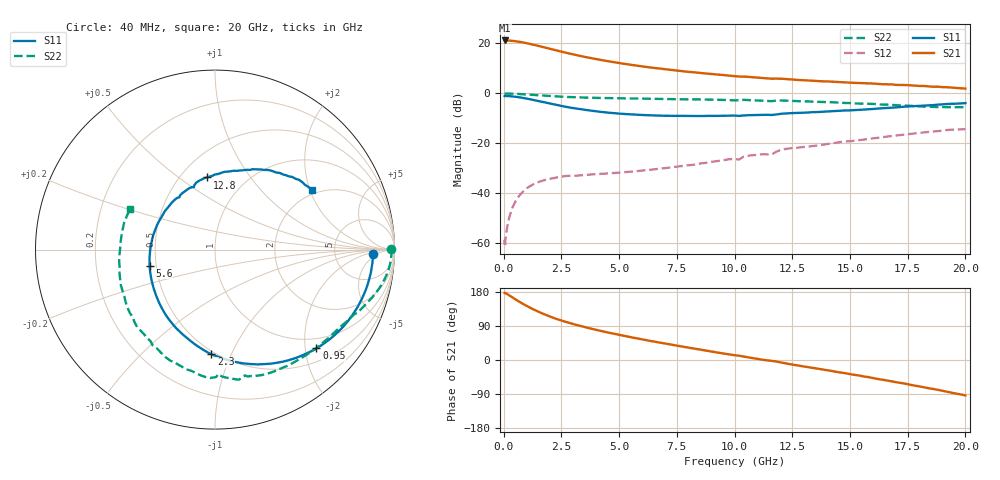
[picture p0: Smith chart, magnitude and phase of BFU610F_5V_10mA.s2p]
! Filename:  P:\Prog\Test\Noise\ATS_data\Testdata_Net\SplitFiles\BFU610_2W_A5_HighFreq_5V_10mA_D.s2p
! Date/Time: Wed 10/Aug/2011 16:58:24
! BFU610_2W_A5_HighFreq_5V_1mA_10mA_Bias4_R.s2p
! MDIF S-parameter v. bias file
! BFU610_2W_A5_HighFreq_5V_1mA_10mA
! Date/time Mon Aug 08 14:15:19 2011
! VAR V_out= 5.0010
! VAR I_out= 9.9950
! VAR V_in= 0.8863
! VAR I_in= 0.0857
! Device data file deembeded for feedlines and parallel
! Original file: \SplitFiles\BFU610_2W_A5_HighFreq_5V_10mA_R.s2p
! Feed-files: PR003V01_101208_Feed1.s2p, PR003V01_101208_Feed2.s2p
! Parallel-file: PR003V01_101208_Par.s2p
# MHz S MA R 50
!  Freq-MHz  S11-mag  S11-arg  S21-mag  S21-arg  S12-mag  S12-arg  S22-mag  S22-arg
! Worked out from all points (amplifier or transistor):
!   167 points, 40 MHz to 20 GHz, reference 50 ohm
!   highest |S21| = 21.1 dB at 40 MHz (marker M1)
!   |S21| within 3 dB of that: start of sweep to 1.861 GHz
!   unconditionally stable (mu >= 1): start of sweep to 59.98 MHz; 3.421 GHz to 17.92 GHz
!   at 550 MHz: K = 0.21, MSG = 31.8 dB, |S12| = -42.7 dB
!   at 4.2 GHz: K = 1.21, MAG = 20.0 dB, |S12| = -32.3 dB
!   at 20 GHz: K = 0.89, MSG = 8.1 dB, |S12| = -14.4 dB
!   S11 on the Smith chart (normalised r, x): 40 MHz: 15, -4; 950 MHz: 0.77, -2.24; 2.3 GHz: 0.48, -0.84; 5.6 GHz: 0.46, -0.10; 12.8 GHz: 0.67, +0.64; 20 GHz: 1.84, +2.06
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40  0.8803 -1.8  11.38 177.2  0.0009164 41.6  0.9799 0.1
50  0.8721 -2.4  11.33 177.4  0.001163 22.7  0.9814 -0.2
140  0.8785 -6.8  11.32 174.4  0.001962 68.5  0.9832 -1.7
260  0.8728 -12.7  11.3 169.7  0.003489 74.4  0.9815 -3.4
400  0.8613 -19.4  11.16 164.2  0.005391 74.8  0.9773 -5.3
650  0.8334 -31.1  10.78 154.8  0.008555 71.0  0.9656 -8.6
950  0.7887 -44.2  10.15 144.2  0.01196 64.8  0.9473 -12.1
1200  0.7482 -54.4  9.569 136.3  0.01433 60.1  0.9302 -14.7
1500  0.6985 -65.8  8.87 127.5  0.01664 55.1  0.9107 -17.6
1850  0.6443 -77.9  8.081 118.3  0.01874 50.4  0.8889 -20.6
2300  0.5826 -92.0  7.139 108.2  0.02065 46.5  0.8619 -24.4
2900  0.5136 -108.4  6.14 96.7  0.02223 40.6  0.8381 -28.1
3400  0.4737 -120.7  5.468 88.6  0.02286 40.3  0.8218 -31.5
4400  0.4142 -142.9  4.468 74.1  0.02465 40.3  0.8014 -37.9
5600  0.3752 -166.2  3.652 59.1  0.02718 43.2  0.7829 -45.9
6800  0.3558 173.0  3.088 45.5  0.03097 46.6  0.7689 -54.0
8800  0.3518 142.7  2.472 24.3  0.04083 50.4  0.7489 -68.2
10200  0.3529 124.1  2.159 11.2  0.04707 52.5  0.7241 -77.0
12800  0.4046 96.2  1.835 -14.9  0.08209 42.5  0.6908 -100.2
13400  0.418 90.2  1.771 -20.8  0.08798 39.6  0.6768 -106.0
16800  0.5153 60.0  1.503 -56.3  0.1392 17.4  0.5848 -146.7
20000  0.6335 31.8  1.238 -93.4  0.1912 -15.4  0.525 154.6
